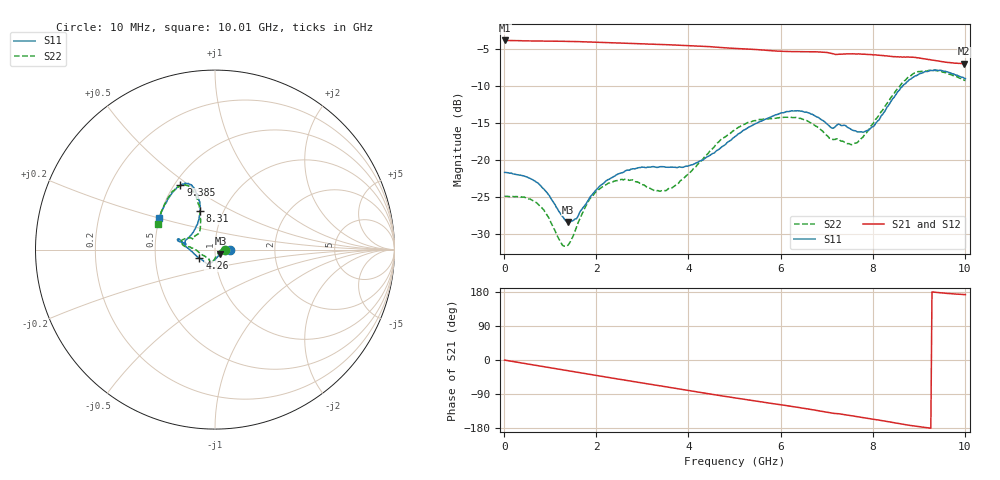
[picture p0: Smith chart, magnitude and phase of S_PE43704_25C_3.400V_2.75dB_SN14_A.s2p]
! Device ID: PE43704
! Dir: z:\PE43704\PE43704_Char_1_20130516\PE43704\AMB\3p400V\2p75dB
! Serial: 14
! Insertion: A
! Impedance: 50 ohm
! Temp: Amb
! VDD: 3.400V
! Attenuation Step: 2.75dB
! IDD: 1.140633e-01mA
#  Hz  S  RI  R  50
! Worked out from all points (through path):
!   401 points, 10 MHz to 10.01 GHz, reference 50 ohm
!   highest |S21| = -3.79 dB at 10 MHz (marker M1); lowest = -6.9 dB at 9.985 GHz (marker M2)
!   group delay of S21, straight-line fit = 53.3 ps
!   lowest |S11| = -28.3 dB at 1.385 GHz (marker M3), VSWR 1.08, Z = 53.1 - j2.48 ohm
!   |S11| at or under -10 dB: start of sweep to 8.642 GHz
!   |S22| runs from -31.6 to -7.8 dB; largest |S21 - S12| = 0.0047
!   S11 on the Smith chart (normalised r, x): 10 MHz: 1.18, +0.00; 4.26 GHz: 0.84, -0.08; 8.31 GHz: 0.78, +0.35; 9.385 GHz: 0.54, +0.46; 10.01 GHz: 0.50, +0.20
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1e7  0.0828 4.61e-05  0.6462 -0.00272  0.6464 -0.00237  0.0571 0.00024
6.85e8  0.0707 0.0127  0.6218 -0.1554  0.6217 -0.1552  0.0495 0.0166
1.235e9  0.0413 -0.012  0.5772 -0.272  0.5772 -0.2718  0.0266 -0.00791
1.385e9  0.0303 -0.0234  0.5605 -0.3017  0.5606 -0.3016  0.0186 -0.0191
1.685e9  0.0102 -0.0455  0.5227 -0.3582  0.5228 -0.3581  0.00366 -0.0428
1.985e9  -0.0071 -0.0622  0.4787 -0.4086  0.4787 -0.4086  -0.00793 -0.0605
2.385e9  -0.0242 -0.074  0.4131 -0.4668  0.4133 -0.4667  -0.0209 -0.0692
3.36e9  -0.0452 -0.0781  0.2302 -0.5622  0.2308 -0.5619  -0.0365 -0.0502
3.735e9  -0.058 -0.068  0.1543 -0.5816  0.1551 -0.5815  -0.0576 -0.0365
4.26e9  -0.0865 -0.0483  0.0464 -0.5894  0.0466 -0.5892  -0.0977 -0.00876
5.01e9  -0.1444 0.00227  -0.0997 -0.5622  -0.0991 -0.5625  -0.1604 0.0162
5.985e9  -0.1995 0.0577  -0.2554 -0.4837  -0.253 -0.484  -0.1898 0.0433
6.685e9  -0.1996 0.0453  -0.3564 -0.408  -0.3566 -0.4073  -0.1667 0.0605
7.085e9  -0.1637 0.0338  -0.4029 -0.3453  -0.4045 -0.3456  -0.1253 0.061
7.585e9  -0.1416 0.0719  -0.4449 -0.2784  -0.4442 -0.278  -0.0889 0.0945
7.96e9  -0.106 0.1275  -0.4711 -0.2164  -0.4712 -0.2178  -0.0807 0.15
8.31e9  -0.0827 0.2133  -0.4841 -0.1552  -0.4825 -0.1568  -0.0875 0.2268
8.36e9  -0.0817 0.2257  -0.4842 -0.1451  -0.4841 -0.147  -0.0875 0.2401
8.835e9  -0.1138 0.3369  -0.494 -0.0596  -0.4909 -0.0614  -0.1406 0.3473
9.385e9  -0.1923 0.3585  -0.4709 0.0126  -0.4716 0.0145  -0.2221 0.3361
9.985e9  -0.305 0.188  -0.4459 0.0564  -0.4479 0.0587  -0.3136 0.1505
1.001e10  -0.3104 0.1761  -0.4475 0.0579  -0.4501 0.059  -0.3165 0.1414
